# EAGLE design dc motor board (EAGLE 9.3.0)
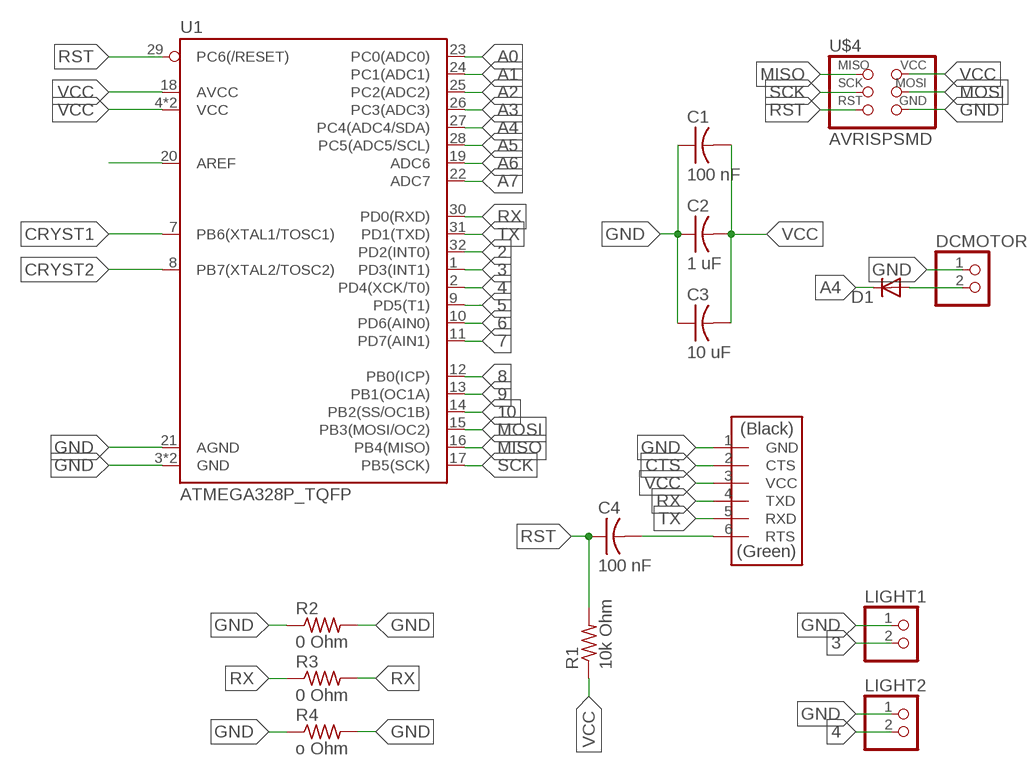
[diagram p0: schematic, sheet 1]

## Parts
C1  100 nF  CAP-US1206FAB  [C1206FAB]
C2  1 uF  CAP-US1206FAB  [C1206FAB]
C3  10 uF  CAP-US1206FAB  [C1206FAB]
C4  100 nF  CAP-US1206FAB  [C1206FAB]
D1  DIODESOD123  [SOD123]
DCMOTOR  PINHD-1X2  [1X02]
LIGHT1  PINHD-1X2  [1X02]
LIGHT2  PINHD-1X2  [1X02]
R1  10k Ohm  RES-US1206FAB  [R1206FAB]
R2  0 Ohm  RES-US1206FAB  [R1206FAB]
R3  0 Ohm  RES-US1206FAB  [R1206FAB]
R4  o Ohm  RES-US1206FAB  [R1206FAB]
U1  ATMEGA328P_TQFP  [TQFP32-08]
U$2  FTDI-SMD-HEADER  [1X06SMD]
U$4  AVRISPSMD  [2X03SMD]

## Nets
2: U1.32(PD2(INT0))
3: LIGHT1.2 U1.1(PD3(INT1))
4: LIGHT2.2 U1.2(PD4(XCK/T0))
5: U1.9(PD5(T1))
6: U1.10(PD6(AIN0))
7: U1.11(PD7(AIN1))
8: U1.12(PB0(ICP))
9: U1.13(PB1(OC1A))
10: U1.14(PB2(SS/OC1B))
A0: U1.23(PC0(ADC0))
A1: U1.24(PC1(ADC1))
A2: U1.25(PC2(ADC2))
A3: U1.26(PC3(ADC3))
A4: D1.CATHODE(C) U1.27(PC4(ADC4/SDA))
A5: U1.28(PC5(ADC5/SCL))
A6: U1.19(ADC6)
A7: U1.22(ADC7)
CRYST1: U1.7(PB6(XTAL1/TOSC1))
CRYST2: U1.8(PB7(XTAL2/TOSC2))
CTS: U$2.2(CTS)
GND: C1.1 C2.1 C3.1 DCMOTOR.1 LIGHT1.1 LIGHT2.1 R2.1 R2.2 R4.1 R4.2 U1.3(GND) U1.5(GND) U1.21(AGND) U$2.1(GND) U$4.6(GND)
MISO: U1.16(PB4(MISO)) U$4.1(MISO)
MOSI: U1.15(PB3(MOSI/OC2)) U$4.4(MOSI)
N$2: D1.ANODE(A) DCMOTOR.2
N$5: U1.20(AREF)
N$7: C4.2 U$2.6(RTS)
RST: C4.1 R1.2 U1.29(PC6(/RESET)) U$4.5(RST)
RX: R3.1 R3.2 U1.30(PD0(RXD)) U$2.4(TXD)
SCK: U1.17(PB5(SCK)) U$4.3(SCK)
TX: U1.31(PD1(TXD)) U$2.5(RXD)
VCC: C1.2 C2.2 C3.2 R1.1 U1.4(VCC) U1.6(VCC) U1.18(AVCC) U$2.3(VCC) U$4.2(VCC)

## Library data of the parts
C1-C4 = fab:CAP-US
D1 = fab:DIODE: DIODE
DCMOTOR LIGHT1 LIGHT2 = pinhead:PINHD-1X2: PIN HEADER
R1-R4 = fab:RES-US: Resistor (US Symbol)
U1 = SparkFun-IC-Microcontroller:ATMEGA328P_TQFP: Popular 328P in QFP Storefront component: ATmega328 - TQFP (COM-13448) Datasheet SparkFun Products SparkFun RedBoard - Programmed with Arduino (DEV-12757) Arduino Pro Mini 328 - 5V/16MHz (DEV-11113) Arduino Pro Mini 328 - 3.3V/8MHz (DEV-11114) SparkFun OpenLog (DEV-13712) SparkFun MicroView - OLED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; PROD_ID: IC-09069
U$2 = fab:FTDI-SMD-HEADER
U$4 = fab:AVRISP

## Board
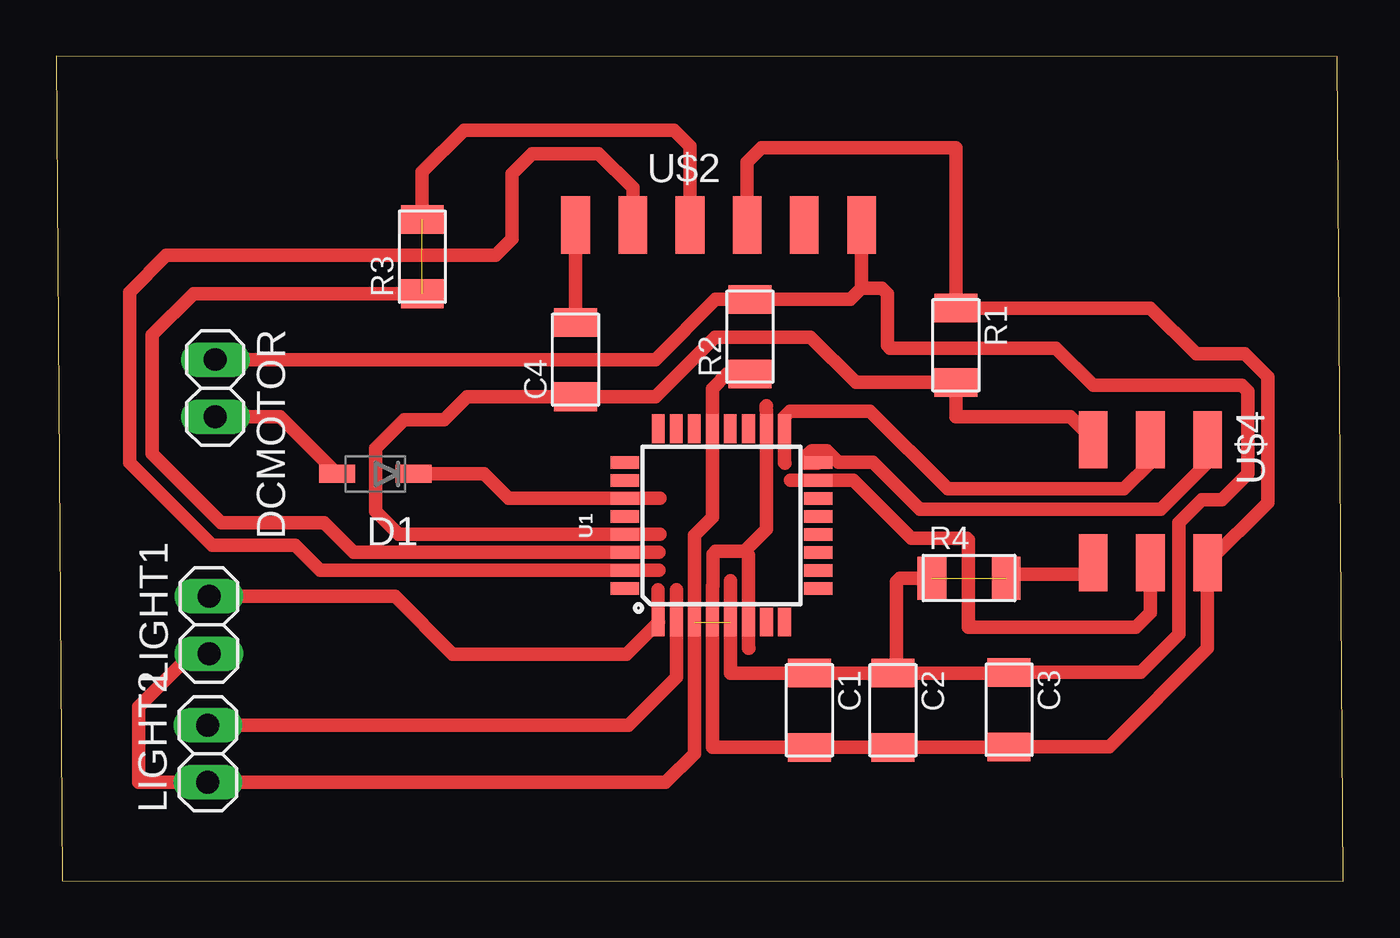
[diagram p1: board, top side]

Size 57.16 x 36.63 mm. Coordinates in mm from the lower left corner, seen from the top.
Outline: 0.25,0.03 57.16,0 56.9,36.6 0,36.63 0.25,0.03
Copper layers (1*16): Top 0.035mm / dielectric 1.5mm / Bottom 0.035mm
Design rules "default *": minimum track width 0.2mm, minimum drill 0.35mm, track to track 6mil, track to pad 6mil, pad to pad 6mil, via to via 6mil, smd to smd 6mil, copper to edge 40mil, drill to drill 6mil, minimum pad ring 10mil, minimum via ring 8mil, stop-mask expansion 4mil, vias tented up to drill 0mil, thermal gap 10mil

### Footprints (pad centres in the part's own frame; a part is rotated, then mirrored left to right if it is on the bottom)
C1206FAB = smd 1.27 x 1.905: 1 -1.651,0; 2 1.651,0
SOD123 = smd 1.6 x 0.8: ANODE 1.7,0; CATHODE -1.7,0
1X02 = drill 1.016 long: 1 -1.27,0; 2 1.27,0
R1206FAB = smd 1.27 x 1.905: 1 -1.651,0; 2 1.651,0
TQFP32-08 = smd 1.27 x 0.559: 1 -4.293,2.8; 2 -4.293,2; 3 -4.293,1.2; 4 -4.293,0.4; 5 -4.293,-0.4; 6 -4.293,-1.2; 7 -4.293,-2; 8 -4.293,-2.8; 17 4.293,-2.8; 18 4.293,-2; 19 4.293,-1.2; 20 4.293,-0.4; 21 4.293,0.4; 22 4.293,1.2; 23 4.293,2; 24 4.293,2.8 | smd 0.559 x 1.27: 9 -2.8,-4.293; 10 -2,-4.293; 11 -1.2,-4.293; 12 -0.4,-4.293; 13 0.4,-4.293; 14 1.2,-4.293; 15 2,-4.293; 16 2.8,-4.293; 25 2.8,4.293; 26 2,4.293; 27 1.2,4.293; 28 0.4,4.293; 29 -0.4,4.293; 30 -1.2,4.293; 31 -2,4.293; 32 -2.8,4.293
1X06SMD = smd 2.54 x 1.27: 1 0,6.35; 2 0,3.81; 3 0,1.27; 4 0,-1.27; 5 0,-3.81; 6 0,-6.35
2X03SMD = smd 2.54 x 1.27: 1 -2.54,2.54; 2 2.92,2.54; 3 -2.54,0; 4 2.92,0; 5 -2.54,-2.54; 6 2.92,-2.54

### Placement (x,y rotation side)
C1  33.45,7.59 270 top
C2  37.16,7.59 270 top
C3  42.32,7.62 270 top
C4  23.06,23.16 90 top
D1  14.17,18.08 180 top
DCMOTOR  7.06,21.89 270 top
LIGHT1  6.78,11.38 90 top
LIGHT2  6.73,5.66 90 top
R1  39.95,23.8 270 top
R2  30.81,24.18 90 top
R3  16.26,27.74 90 top
R4  40.54,13.46 0 top
U1  29.54,15.8 90 top
U$2  29.41,29.13 270 top
U$4  48.59,17.07 270 top

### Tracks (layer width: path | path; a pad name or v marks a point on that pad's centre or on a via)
3
  Top 0.61: LIGHT1.2 15.04,12.65 17.6,10.08 25.32,10.08 U1.1 26.72,11.53 26.72,12.95
4
  Top 0.61: LIGHT2.2 25.41,6.93 27.54,9.07 U1.2 27.54,12.95
A4
  Top 0.61: D1.CATHODE 19,18.08 20.09,17 U1.27 26.8,17
GND  (2 unrouted)
  Top 0.61: C2.1 C1.1 29.94,9.25 U1.5 29.94,13.34 | LIGHT2.1 5.97,4.39 | LIGHT2.1 27.06,4.39 28.34,5.67 U1.3 28.34,15.36 29.14,16.16 U1.21 29.14,21.88 29.79,22.53 R2.1 | U$2.1 35.76,26.33 | 35.76,26.33 35.27,25.83 R2.2 29.29,25.83 26.62,23.16 DCMOTOR.1 | 35.76,26.33 36.66,26.33 36.91,26.09 36.91,23.8 37.03,23.67 44.4,23.67 46.05,22.02 52.65,22.02 52.91,21.77 52.91,18.08 51.77,16.94 50.88,16.94 49.86,15.93 49.86,10.97 48.16,9.27 C3.1 42.29,9.25 C2.1 | LIGHT1.1 6.02,10.11 3.66,7.75 3.66,4.39 LIGHT2.1 | C2.1 37.31,9.4 37.31,13.31 37.47,13.46 R4.1 | R4.2 42.37,13.64 45.54,13.64 U$4.6
MISO
  Top 0.61: U$4.1 51.13,18.59 49.05,16.51 38.35,16.51 36.27,18.6 34.75,18.6 34.22,19.13 33.55,19.13 33.27,18.85 33.27,18.57 33.8,18.57 U1.16
MOSI
  Top 0.61: 32.61,17.8 U1.15 35.41,17.8 37.97,15.24 40.44,15.24 40.51,15.16 40.51,11.28 47.96,11.28 48.59,11.91 U$4.4
N$2
  Top 0.61: D1.ANODE 9.93,20.62 DCMOTOR.2
N$7
  Top 0.61: C4.2 U$2.6
RST
  Top 0.61: U$4.5 45.03,20.62 39.95,20.62 R1.2 35.51,22.15 33.5,24.16 29.26,24.16 26.62,21.51 C4.1 18.24,21.51 17.22,20.5 15.44,20.5 14.17,19.23 14.17,16.43 15.21,15.4 U1.29 26.8,15.4
RX  (1 unrouted)
  Top 0.61: 28.02,29.01 U$2.4 28.14,32.64 27.43,33.35 18.11,33.35 16.26,31.5 R3.2 | R3.1 6.1,26.09 4.27,24.26 4.27,18.97 7.32,15.93 11.89,15.93 13.21,14.6 U1.30 26.76,14.6
SCK
  Top 0.61: U$4.3 48.59,18.59 47.42,17.42 39.6,17.42 36.14,20.88 32.59,20.88 32.34,20.63 U1.17 32.34,18.58 32.36,18.56
TX
  Top 0.61: U$2.5 25.6,30.78 24.08,32.31 21.13,32.31 20.24,31.42 20.24,28.52 19.51,27.79 4.88,27.79 3.25,26.16 3.25,18.59 6.93,14.91 10.62,14.91 11.73,13.8 U1.31 26.77,13.8
VCC
  Top 0.61: 30.56,14.66 29.29,14.66 29.16,14.53 29.16,13.13 29.14,13.11 U1.4 29.14,5.94 C1.2 C2.2 42.29,5.94 C3.2 46.76,5.97 51.13,10.34 U$4.2 53.8,16.82 53.8,22.4 52.78,23.42 50.62,23.42 48.59,25.45 R1.1 39.95,32.56 31.32,32.56 30.68,31.93 U$2.3 | 30.56,14.66 30.74,14.47 U1.6 30.74,10.36 30.76,10.34 | 30.56,14.66 31.54,15.64 U1.18 31.54,20.91 31.52,20.93 31.52,21.08 31.55,21.11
